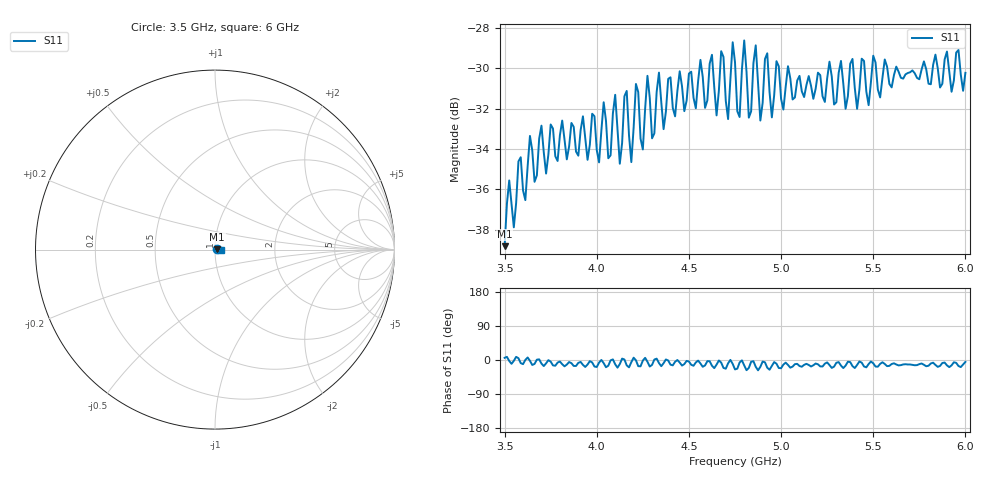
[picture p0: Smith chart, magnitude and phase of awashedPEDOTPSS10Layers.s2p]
!  31/07/2025  11:01:13
! Ref Plane: 0.000 mm
# MHZ S MA R  50
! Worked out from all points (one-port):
!   201 points, 3.5 GHz to 6 GHz, reference 50 ohm
!   lowest |S11| = -38.8 dB at 3.5 GHz (marker M1), VSWR 1.02, Z = 51.2 + j0.117 ohm
!   |S11| at or under -10 dB: start of sweep to end of sweep
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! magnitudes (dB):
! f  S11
! 3.5 GHz  -38.8
! 3.525 GHz  -35.6
! 3.55 GHz  -37.9
! 3.638 GHz  -33.4
! 3.812 GHz  -32.6
! 4.013 GHz  -34.7
! 4.037 GHz  -31.7
! 4.062 GHz  -34.5
! 4.1 GHz  -31.3
! 4.125 GHz  -34.7
! 4.162 GHz  -31.1
! 4.188 GHz  -34.7
! 4.213 GHz  -30.8
! 4.25 GHz  -34.0
! 4.275 GHz  -30.4
! 4.3 GHz  -33.5
! 4.338 GHz  -30.2
! 4.362 GHz  -33.0
! 4.438 GHz  -31.1
! 4.625 GHz  -29.3
! 4.65 GHz  -32.3
! 4.675 GHz  -29.2
! 4.713 GHz  -32.5
! 4.75 GHz  -29.7
! 5.062 GHz  -31.6
! 5.375 GHz  -29.8
! 5.688 GHz  -30.2
! 6 GHz  -30.2
